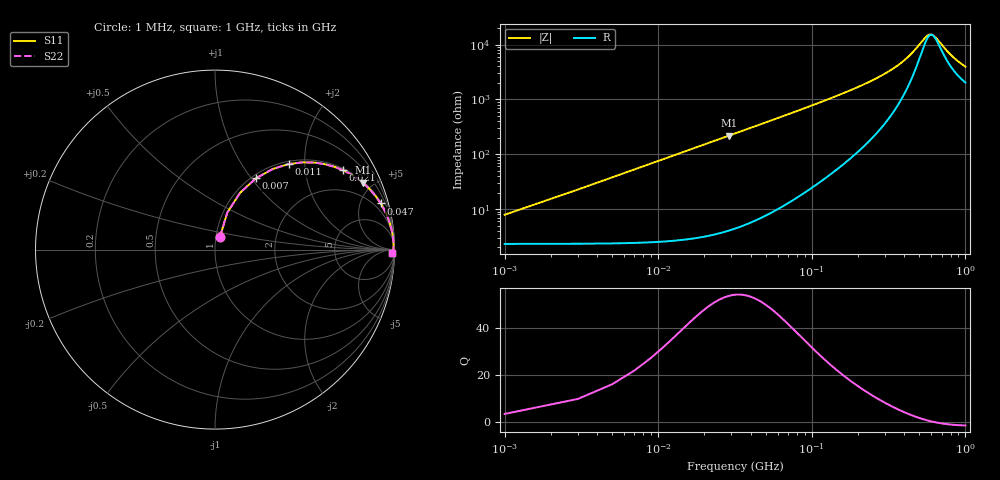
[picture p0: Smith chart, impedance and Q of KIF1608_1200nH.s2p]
# MHz S RI R 50
!Freq ReS11 ImS11 ReS21 ImS21 ReS12 ImS12 ReS22 ImS22
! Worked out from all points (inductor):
!   501 points, 1 MHz to 1 GHz, reference 50 ohm
!   read as one part in series: L = 1.2 uH near 5 MHz
!   highest Q = 53.6 at 29 MHz (marker M1), where L = 1.2 uH
!   self-resonance near 606.2 MHz
!   S11 on the Smith chart (normalised r, x): 1 MHz: 1.05, +0.15; 7 MHz: 1.05, +1.06; 11 MHz: 1.05, +1.66; 21 MHz: 1.06, +3.17; 47 MHz: 1.14, +7.13; 1 GHz: 42, -68
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1  0.0279 0.0716  0.9721 -0.0716  0.9721 -0.0716  0.0279 0.0716
3  0.0683 0.2059  0.9317 -0.2059  0.9317 -0.2059  0.0683 0.2059
7  0.2285 0.3976  0.7715 -0.3976  0.7715 -0.3976  0.2285 0.3976
9  0.3217 0.4492  0.6783 -0.4492  0.6783 -0.4492  0.3217 0.4492
11  0.4106 0.4767  0.5894 -0.4767  0.5894 -0.4767  0.4106 0.4767
15  0.5601 0.4842  0.4399 -0.4842  0.4399 -0.4842  0.5601 0.4842
21  0.7114 0.443  0.2886 -0.443  0.2886 -0.443  0.7114 0.443
29  0.8231 0.3724  0.1769 -0.3724  0.1769 -0.3724  0.8231 0.3724
47  0.9227 0.2574  0.0773 -0.2574  0.0773 -0.2574  0.9227 0.2574
69  0.9612 0.1816  0.0388 -0.1816  0.0388 -0.1816  0.9612 0.1816
95  0.9779 0.1327  0.0221 -0.1327  0.0221 -0.1327  0.9779 0.1327
169  0.9909 0.0716  0.00906 -0.0716  0.00906 -0.0716  0.9909 0.0716
335  0.9949 0.0274  0.00508 -0.0274  0.00508 -0.0274  0.9949 0.0274
423  0.9949 0.016  0.00511 -0.016  0.00511 -0.016  0.9949 0.016
501  0.9944 0.00831  0.00556 -0.00831  0.00556 -0.00831  0.9944 0.00831
551  0.994 0.00413  0.006 -0.00413  0.006 -0.00413  0.994 0.00413
585  0.9936 0.00153  0.00635 -0.00153  0.00635 -0.00153  0.9936 0.00153
619  0.9933 -0.0009  0.00675 0.0009  0.00675 0.0009  0.9933 -0.0009
667  0.9926 -0.00409  0.00737 0.00409  0.00737 0.00409  0.9926 -0.00409
751  0.9914 -0.00912  0.00863 0.00912  0.00863 0.00912  0.9914 -0.00912
835  0.9899 -0.0136  0.0101 0.0136  0.0101 0.0136  0.9899 -0.0136
1000  0.9867 -0.0211  0.0133 0.0211  0.0133 0.0211  0.9867 -0.0211
